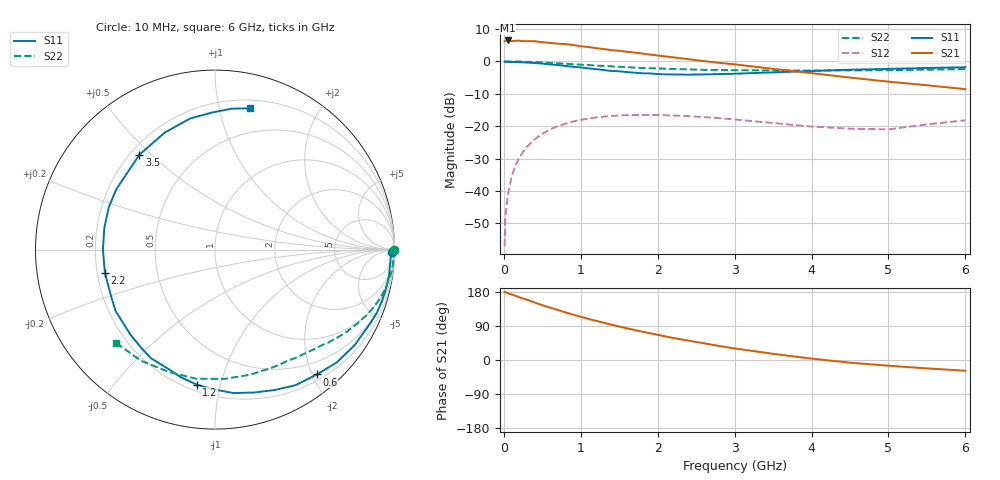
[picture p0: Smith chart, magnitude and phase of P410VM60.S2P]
! SIEMENS Small Signal Semiconductors
! BFP182
! Si NPN RF Bipolar Junction Transistor in SOT143
! VCE = 10 V  IC = 0.6 mA
! Common Emitter S-Parameters:  March  1996
# GHz  S  MA  R  50
!  f  S11  S21  S12  S22
! GHz  MAG  ANG  MAG  ANG  MAG  ANG  MAG  ANG
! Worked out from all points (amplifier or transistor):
!   36 points, 10 MHz to 6 GHz, reference 50 ohm
!   highest |S21| = 6.5 dB at 50 MHz (marker M1)
!   |S21| within 3 dB of that: start of sweep to 1.405 GHz
!   unconditionally stable (mu >= 1): 2.871 GHz to end of sweep
!   at 250 MHz: K = 0.10, MSG = 17.1 dB, |S12| = -27.9 dB
!   at 1.4 GHz: K = 0.51, MSG = 10.2 dB, |S12| = -16.9 dB
!   at 6 GHz: K = 1.19, MAG = 2.1 dB, |S12| = -18.2 dB
!   S11 on the Smith chart (normalised r, x): 10 MHz: open; 600 MHz: 0.29, -2.07; 1.2 GHz: 0.24, -0.84; 2.2 GHz: 0.23, -0.10; 3.5 GHz: 0.24, +0.46; 6 GHz: 0.27, +1.25
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0.01  0.9877 -0.9  2.052 179.6  0.0014 84.8  0.999 -0.2
0.02  0.9808 -1.7  2.084 179.3  0.0039 81.7  0.9999 -0.7
0.05  0.979 -4.4  2.104 176.5  0.0083 87.6  0.9979 -1.6
0.1  0.9804 -8.6  2.053 173.0  0.0165 84.5  0.994 -3.2
0.15  0.977 -13.1  2.083 169.4  0.0246 81.0  0.9945 -4.8
0.25  0.9679 -21.4  2.047 162.2  0.0401 75.5  0.9889 -8.0
0.4  0.9427 -34.3  2.047 151.6  0.0624 67.3  0.9753 -12.5
0.6  0.8978 -50.8  1.931 138.4  0.0889 56.7  0.9497 -18.2
0.8  0.8503 -66.9  1.848 125.7  0.109 47.0  0.9201 -23.4
0.9  0.8253 -74.8  1.791 119.7  0.118 42.4  0.9034 -25.7
1.1  0.7786 -90.7  1.667 108.4  0.1311 34.1  0.8752 -30.2
1.2  0.7591 -97.8  1.601 103.4  0.1362 29.9  0.8628 -32.4
1.5  0.7027 -120.4  1.46 88.2  0.1457 20.0  0.8246 -37.9
1.7  0.6681 -134.8  1.366 79.2  0.1481 14.2  0.8011 -41.4
2.2  0.6271 -167.9  1.155 58.2  0.146 2.1  0.7631 -49.7
2.8  0.637 158.3  0.948 37.0  0.1331 -7.9  0.7354 -60.2
3.5  0.6761 128.5  0.766 16.3  0.1116 -12.7  0.7241 -74.3
4  0.7098 113.2  0.658 3.7  0.0984 -10.0  0.7223 -85.7
4.5  0.7438 100.6  0.562 -7.1  0.0913 -4.2  0.7269 -98.1
5  0.7645 91.0  0.486 -15.1  0.0891 7.8  0.7287 -110.7
5.5  0.7912 83.1  0.428 -22.2  0.1065 13.6  0.7442 -123.8
6  0.8114 75.9  0.372 -28.3  0.1231 14.8  0.7577 -136.6
